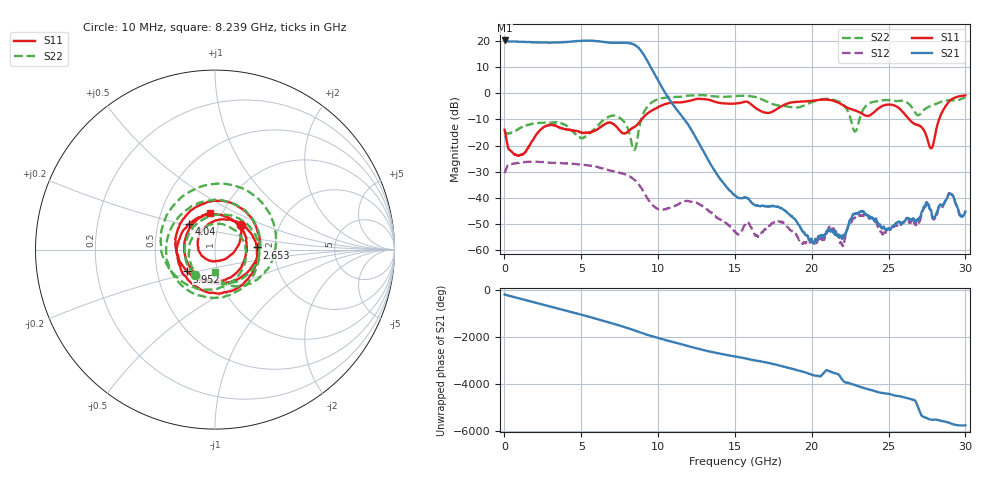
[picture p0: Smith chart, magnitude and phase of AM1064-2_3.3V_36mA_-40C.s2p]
!Agilent	"Technologies,E8364B,MY43040894,A.07.50.67"
!Agilent	E8364B:	A.07.50.67
!Date:	"Wednesday,"	May	"01,"	2019	6:26:02
!Correction:	S11(Full	2	"Port(1,2))"
!S21(Full	2	"Port(1,2))"
!S12(Full	2	"Port(1,2))"
!S22(Full	2	"Port(1,2))"
!S2P	File:	Measurements:	"S11,"	"S21,"	"S12,"	S22:
#	Hz	S	dB	R	50
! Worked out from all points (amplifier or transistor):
!   1601 points, 10 MHz to 30 GHz, reference 50 ohm
!   highest |S21| = 20.1 dB at 10 MHz (marker M1)
!   |S21| within 3 dB of that: start of sweep to 8.754 GHz
!   unconditionally stable (mu >= 1): start of sweep to end of sweep
!   at 4.996 GHz: K = 1.35, MAG = 20.1 dB, |S12| = -27.3 dB
!   at 15.01 GHz: K = 2842.28, MAG = -30.6 dB, |S12| = -52.9 dB
!   at 30 GHz: K = 942.07, MAG = -32.9 dB, |S12| = -45.0 dB
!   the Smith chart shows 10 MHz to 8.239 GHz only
!   S11 on the Smith chart (normalised r, x): 10 MHz: 1.28, +0.37; 2.653 GHz: 1.60, +0.04; 4.04 GHz: 0.72, +0.21; 5.952 GHz: 0.71, -0.18; 8.239 GHz: 0.87, +0.37
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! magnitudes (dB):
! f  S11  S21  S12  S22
! 10 MHz  -14.0  20.1  -30.5  -14.9
! 1.003 GHz  -23.6  19.6  -26.5  -13.4
! 2.653 GHz  -12.7  19.3  -26.4  -11.2
! 4.04 GHz  -13.8  19.5  -26.8  -12.5
! 5.015 GHz  -15.0  19.9  -27.3  -17.2
! 5.952 GHz  -14.1  19.9  -28.1  -13.1
! 7.301 GHz  -12.9  19.2  -30.1  -8.8
! 8.239 GHz  -13.7  18.9  -32.1  -17.9
! 8.482 GHz  -12.8  18.4  -33.2  -21.5
! 10.02 GHz  -5.3  4.5  -44.2  -2.3
! 12.46 GHz  -2.3  -17.0  -41.8  -0.8
! 15.01 GHz  -4.0  -39.1  -52.9  -1.2
! 17.85 GHz  -5.6  -43.5  -49.0  -4.7
! 20.01 GHz  -2.9  -56.8  -56.6  -3.5
! 21.23 GHz  -2.7  -52.9  -51.1  -2.3
! 21.98 GHz  -4.4  -55.6  -57.8  -4.0
! 22.82 GHz  -6.6  -46.0  -47.4  -14.6
! 23.59 GHz  -8.7  -46.6  -47.3  -4.5
! 25.01 GHz  -4.3  -51.9  -51.6  -2.7
! 27.77 GHz  -21.1  -44.7  -44.8  -4.8
! 28.74 GHz  -4.7  -40.8  -40.7  -2.8
! 30 GHz  -0.9  -45.2  -45.0  -1.7
